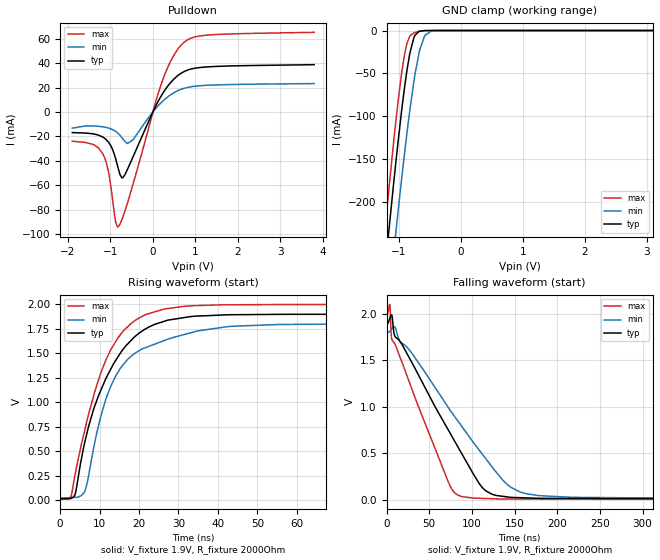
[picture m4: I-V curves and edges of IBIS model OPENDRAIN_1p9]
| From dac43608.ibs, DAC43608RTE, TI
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|   OPENDRAIN_1p9 Model
[Model]   OPENDRAIN_1p9
Model_type   I/O_open_drain
Polarity   Non-Inverting
Enable   Active-Low
Vinl = 0.5
Vinh = 1.6
Vmeas = 0.95
Vref = 1.9
Cref = 2pF
Rref = 2000
|   typ   min   max
C_comp   1.246E-12   1.224E-12   1.275E-12
|  Where Nom  PVT is Nominal Process, 1.9V,   25C
|   Fast PVT is Strong Process,  2.0V,  -40C
|   Slow PVT is Weak Process,   1.8V,  125C
[Voltage Range]   1.9   1.8   2
|Junction Temperature
[Temperature Range]   25   125   -40
[Pullup Reference]   1.9   1.8   2
[Pulldown Reference]   0   0   0
[Power Clamp Reference]   1.9   1.8   2
[GND Clamp Reference]   0   0   0
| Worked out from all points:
|   slope of the pulldown table from 0 to 0.285 V, typ, clamps not added: 15.8 ohm
|   GND clamp passes 1 mA (typ) near -0.68 V on its own axis
|   falling waveform, V_fixture 1.9V, R_fixture 2000Ohm: 20-80 % time 67.9ns typ, 82.2ns min, 50.2ns max; typ from 1.9 V to 0.013 V
|   rising waveform, V_fixture 1.9V, R_fixture 2000Ohm: 20-80 % time 10.4ns typ, 9.46ns min, 9.26ns max; typ from 0.013 V to 1.9 V
[Pulldown]
|   Voltage   I(typ)   I(min)   I(max)
-1.9V     -16.87mA   -13.27mA   -23.93mA
-1.182V   -20.5mA    -12.14mA   -34.13mA
-1.045V   -24.77mA   -13.19mA   -49.25mA
-891.1mV  -36.58mA   -15.58mA   -87.45mA
-828.4mV  -44.67mA   -17.21mA   -94.23mA
-731.5mV  -53.86mA   -20.95mA   -88.1mA
-657.4mV  -51.18mA   -24.17mA   -80.86mA
-469.3mV  -36.8mA    -22.78mA   -59.23mA
191.9mV   12.92mA    7.52mA     22.34mA
722mV     32.84mA    19.23mA    56.63mA
1.286V    36.88mA    21.84mA    62.87mA
3.8V      38.68mA    23.23mA    65.15mA
[GND Clamp]
|   Voltage   I(typ)   I(min)   I(max)
-1.9V     -800.6mA   -857.2mA   -767.4mA
-1.233V   -283.4mA   -363.5mA   -236.2mA
-1.193V   -254mA     -334.8mA   -206.2mA
-1.056V   -157mA     -238.6mA   -109mA
-1.022V   -134.1mA   -215.4mA   -86.94mA
-908.2mV  -65.02mA   -141.5mA   -27.18mA
-828.4mV  -27.86mA   -94.59mA   -6.905mA
-760mV    -8.358mA   -59.35mA   -2.79mA
-668.8mV  -833uA     -23.67mA   -793.5uA
-583.3mV  -106.4uA   -5.689mA   -134.7uA
-469.3mV  -5.674uA   -327.9uA   -5.529uA
3.8V      0A         0A         0A
[POWER Clamp]
|   Voltage   I(typ)   I(min)   I(max)
-1.9V     0A         0A         0A
0V        0A         0A         0A
3.8V      0A         0A         0A
[Ramp]
R_load = 2000
|   typ   min   max
dV/dt_r   1.13247/1.03727e-08   1.06762/9.46382e-09   1.19545/9.22387e-09
dV/dt_f   1.13247/6.80025e-08   1.06762/8.2166e-08   1.19545/5.03103e-08
[Falling Waveform]
V_fixture = 1.9V
V_fixture_min = 1.8V
V_fixture_max = 2V
R_fixture = 2000Ohm
C_fixture = 0F
|   Time   V(typ)   V(min)   V(max)
0s        1.9V       1.8V       2V
3.764ns   1.953V     1.812V     2.1V
5.274ns   1.986V     1.831V     1.792V
6.297ns   1.976V     1.844V     1.719V
9.88ns    1.755V     1.857V     1.671V
72.48ns   749.4mV    991.9mV    190.6mV
83.93ns   565.2mV    843.7mV    51.8mV
116.8ns   96.23mV    437.5mV    16.33mV
163.7ns   23mV       68.03mV    11.09mV
500ns     12.55mV    20.63mV    7.587mV
[Rising Waveform]
V_fixture = 1.9V
V_fixture_min = 1.8V
V_fixture_max = 2V
R_fixture = 2000Ohm
C_fixture = 0F
|   Time   V(typ)   V(min)   V(max)
0s        12.55mV    20.63mV    7.587mV
2.553ns   16.71mV    25.45mV    19.46mV
3.738ns   53.02mV    27.68mV    250mV
6.295ns   600.1mV    94.22mV    724.3mV
10.23ns   1.115V     844.9mV    1.291V
14.49ns   1.454V     1.296V     1.649V
21.19ns   1.74V      1.552V     1.887V
31.52ns   1.867V     1.694V     1.982V
71.82ns   1.9V       1.8V       2V
500ns     1.9V       1.8V       2V
